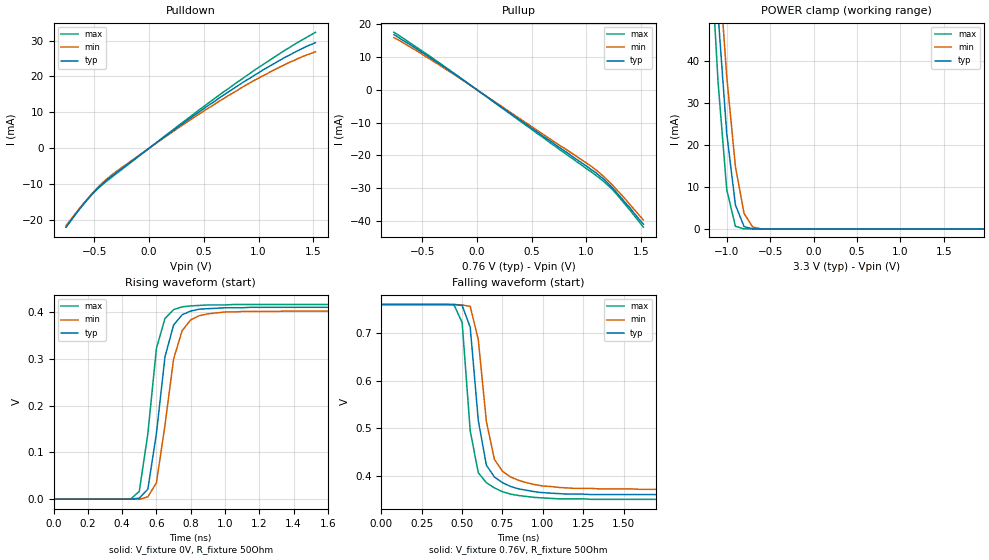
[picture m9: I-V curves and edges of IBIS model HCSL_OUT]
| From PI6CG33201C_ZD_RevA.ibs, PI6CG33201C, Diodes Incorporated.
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[Model]  HCSL_OUT
Model_type  Output
Vmeas =  0.2
Vref = 0
Rref = 50
|Variable   typ   min   max
C_comp   1.41p   1.40p  1.42p
|Variable   typ   min   max
[Voltage Range]   0.76   0.76   0.76
[Temperature Range]   25   85   -40
[POWER Clamp Reference]   3.3   3.135   3.465
[Pullup Reference]   0.76   0.76   0.76
[Pulldown Reference]   0   0   0
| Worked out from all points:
|   slope of the pulldown table from 0 to 0.114 V, typ, clamps not added: 44.1 ohm
|   slope of the pullup table from 0 to 0.114 V, typ, clamps not added: 42.4 ohm
|   POWER clamp passes 1 mA (typ) near -0.81 V on its own axis
|   falling waveform, V_fixture 0.76V, R_fixture 50Ohm: 20-80 % time 82.6ps typ, 89.6ps min, 75.6ps max; typ from 0.76 V to 0.359 V
|   rising waveform, V_fixture 0V, R_fixture 50Ohm: 20-80 % time 92.1ps typ, 100ps min, 81.2ps max; typ from 0 V to 0.411 V
[Power clamp]
| Voltage   I(typ)   I(min)  I(max)
-3.3V     1.02A      977mA      1.08A
-1.2V     86.3mA     99mA       71.7mA
-1.1V     51.3mA     65.5mA     35.1mA
-1V       22.8mA     36.4mA     9.39mA
-900mV    5.72mA     14.9mA     638uA
-800mV    544uA      3.68mA     8.25uA
-700mV    18.7uA     441uA      62.5nA
-600mV    428nA      26.6uA     447pA
6.6V      -19.8pA    -19.9pA    -19.8pA
[Pulldown]   |Note: Vtable = Vcc - Voutput
| Voltage   I(typ)   I(min)  I(max)
-760mV    -22mA      -21.6mA    -22mA
-600mV    -15.6mA    -15.4mA    -15.6mA
-520mV    -12.7mA    -12.6mA    -12.8mA
-440mV    -10.3mA    -10mA      -10.5mA
-320mV    -7.26mA    -6.93mA    -7.57mA
80mV      1.82mA     1.72mA     1.9mA
520mV     11.5mA     10.8mA     12.1mA
960mV     20.3mA     18.9mA     21.7mA
1.24V     25.3mA     23.3mA     27.3mA
1.44V     28.4mA     26mA       30.9mA
1.52V     29.4mA     26.9mA     32.3mA
[Pullup]   |Note: Vtable = Vcc - Voutput
| Voltage   I(typ)   I(min)  I(max)
-760mV    16.9mA     16mA       17.6mA
-520mV    11.8mA     11.3mA     12.3mA
-200mV    4.67mA     4.46mA     4.83mA
1.04V     -24.3mA    -23.3mA    -25mA
1.16V     -27.4mA    -26.6mA    -28.1mA
1.24V     -30.1mA    -29.2mA    -30.6mA
1.4V      -36.2mA    -35.2mA    -36.9mA
1.52V     -41.1mA    -39.8mA    -42mA
[Falling Waveform]
V_fixture = 0.76V
V_fixture_min = 0.76V
V_fixture_max = 0.76V
R_fixture = 50Ohm
C_fixture = 0F
|   Time   V(typ)   V(min)   V(max)
0s        760mV      760mV      760mV
450ps     760mV      760mV      759mV
500ps     758mV      759mV      722mV
550ps     712mV      756mV      494mV
600ps     516mV      686mV      406mV
650ps     422mV      514mV      385mV
700ps     397mV      434mV      374mV
800ps     377mV      397mV      361mV
1.35ns    360mV      372mV      350mV
4.95ns    359mV      371mV      350mV
[Rising Waveform]
V_fixture = 0V
V_fixture_min = 0V
V_fixture_max = 0V
R_fixture = 50Ohm
C_fixture = 0F
|   Time   V(typ)   V(min)   V(max)
0s        0V         0V         0V
450ps     -51.3uV    -107uV     534uV
500ps     2.12mV     -351uV     16.6mV
550ps     21.6mV     4.94mV     140mV
600ps     141mV      35mV       323mV
650ps     305mV      159mV      387mV
700ps     373mV      300mV      406mV
750ps     395mV      361mV      412mV
1ns       410mV      401mV      416mV
4.95ns    411mV      403mV      417mV
[Ramp]
|   typ   min   max
dV/dt_r   0.247/0.08E-12   0.246/0.09E-12   0.248/0.07E-12
dV/dt_f   0.240/0.07E-12   0.239/0.08E-12   0.241/0.06E-12
R_load =   50.0000
